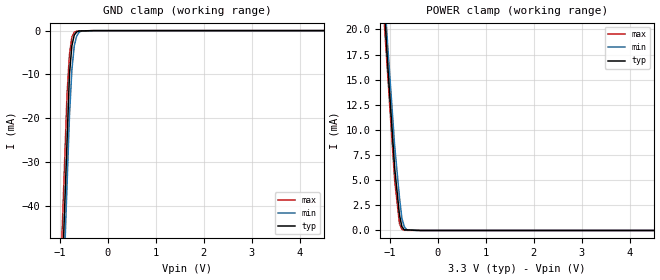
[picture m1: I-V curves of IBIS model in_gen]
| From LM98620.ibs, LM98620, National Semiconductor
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[Model] in_gen
Model_type Input
Vinl = 800.000mV
Vinh = 2.00000V
C_comp 1.23000pF 1.19000pF 1.31000pF
| variable typ   min   max
[Voltage Range] 3.30000V 3.00000V 3.60000V
[POWER Clamp Reference] 3.30000V 3.00000V 3.60000V
[GND Clamp Reference] 0.00000V 0.00000V 0.00000V
[Temperature Range]   25   70   0
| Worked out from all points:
|   GND clamp passes 1 mA (typ) near -0.70 V on its own axis
|   POWER clamp passes 1 mA (typ) near -0.78 V on its own axis
[GND Clamp]
-3.3V     -772.6mA   -803.8mA   -764mA
-850mV    -25.17mA   -35.14mA   -14.33mA
-800mV    -9.917mA   -19.45mA   -5.347mA
-750mV    -3.457mA   -9.001mA   -1.497mA
-700mV    -994.8uA   -3.453mA   -369.7uA
-650mV    -301.2uA   -1.25mA    -102.1uA
-600mV    -79.92uA   -375.7uA   -87.1uA
-550mV    -67.53uA   -111.6uA   -72.13uA
-325mV    -11.81uA   -22.71uA   -4.778uA
-300mV    -5.623uA   -12.84uA   -4.746uA
-275mV    -5.571uA   -2.966uA   -4.713uA
6.6V      8.676uA    4.259uA    4.17uA
[POWER Clamp]
-3.3V     204mA      183.1mA    179mA
-1.15V    25.18mA    26.05mA    23.1mA
-1.1V     21.02mA    22.4mA     19.47mA
-1.05V    16.86mA    18.75mA    15.85mA
-900mV    6.209mA    8.408mA    4.971mA
-800mV    1.526mA    3.293mA    663.9uA
-750mV    388.7uA    1.214mA    114.4uA
-700mV    67.35uA    378uA      16.6uA
-650mV    57.73uA    78.46uA    14.94uA
-450mV    19.24uA    0A         8.301uA
6.6V      0A         0A         0A
